| TI TMS320DM365 ZCE IBIS MODEL
[IBIS Ver]   4.0
[File Name]   sprm354.ibs
[File Rev]   1.02
[Date]   August 12, 2010
[Source]   From silicon level SPICE model at Texas Instruments Inc.,
[Notes]   -RevA   Added DDR IBIS info.
		-RevB 	Updated/fixed DDR IBIS info.
   -RevC   Remove a unnecessary note.
[Disclaimer] Please be aware that in the absence of a written agreement,
   Texas Instruments (TI) assumes no liability for: 1) the
   accuracy of the IBIS models provided to your company, 2) the
   proper functioning of these IBIS models in your design or for
   any resulting applications, or; 3) infringement of patents,
   copyrights, or intellectual property rights resulting from
   your use of these IBIS models. TI provides IBIS models as a
   service to our customers and therefore reserves the right to
   limit distribution of the IBIS models.
[Copyright]   Property of Texas Instruments Incorporated. Unauthorized
   reproduction and/or distribution is strictly prohibited. This
   product is protected under copyright law and trade secret law
   as an unpublished work. Copyright (C) 2008, Texas Instruments
   Incorporated, all rights reserved. These commodities are under
   the U.S. Government distribution license control. As such,
   they are not to be re-exported without the prior approval of
   the U.S. Department of Commerce.
| Component   DM365
[Component]   DM365
[Manufacturer]   Texas Instruments
[Package]
| variable   typ   min   max
R_pkg   2.50E-01   2.85E-03   3.42E-01
L_pkg   3.37E-09   8.62E-11   5.01E-09
C_pkg   9.39E-13   4.32E-13   3.43E-11
[Pin] signal_name   model_name   R_pin   L_pin   C_pin
W19   VSS   GND   2.85E-03   8.62E-11   3.43E-11
A1   RSV0   NC   2.88E-01   4.46E-09   4.90E-13
E5   VDD18_SLD0   POWER   5.60E-02   1.13E-09   7.80E-13
D4   VDDRAM   NC   2.37E-01   3.20E-09   7.66E-13
B3   GIO6   BC1833DV65ATHYPBFZP   2.43E-01   3.73E-09   7.84E-13
H6   VDDS33   POWER   8.08E-03   1.69E-10   1.01E-11
A3   GIO7   BC1833DV65ATHYPBFZP   3.13E-01   4.61E-09   8.76E-13
A2   GIO8   BC1833DV65ATHYPBFZP   3.06E-01   4.77E-09   6.55E-13
C2   GIO9   BC1833DV65ATHYPBFZP   2.29E-01   3.51E-09   8.41E-13
B2   GIO10   BC1833DV65ATHYPBFZP   3.19E-01   4.70E-09   7.26E-13
G6   CVDD   POWER   5.00E-03   1.20E-10   2.07E-11
B1   GIO11   BC1833DV65ATHYPBFZP   3.18E-01   4.90E-09   5.92E-13
C1   GIO12   BC1833DV65ATHYPBFZP   2.88E-01   4.22E-09   5.60E-13
D3   GIO13   BC1833DV65ATHYPBFZP   2.21E-01   3.18E-09   7.81E-13
D1   GIO14   BC1833DV65ATHYPBFZP   2.85E-01   4.00E-09   4.66E-13
D2   GIO15   BC1833DV65ATHYPBFZP   2.85E-01   3.85E-09   5.44E-13
E1   GIO16   BC1833DV65ATHYPBFZP   2.36E-01   3.69E-09   5.56E-13
E4   GIO17   BC1833DV65ATHYPBFZP   2.26E-01   3.16E-09   6.86E-13
E2   GIO18   BC1833DV65ATHYPBFZP   2.99E-01   3.96E-09   6.09E-13
E3   GIO19   BC1833DV65ATHYPBFZP   2.97E-01   3.86E-09   6.67E-13
F1   GIO20   BC1833DV65ATHYPBFZP   2.76E-01   4.04E-09   6.21E-13
F3   GIO21   BC1833DV65ATHYPBFZP   2.19E-01   2.93E-09   6.69E-13
F2   RTCK   BC1833DV65ATHYPBFZP   2.63E-01   3.42E-09   5.45E-13
F4   TCK   BC1833DV65ATHYPBFZP   2.31E-01   3.14E-09   7.64E-13
F5   TDI   BC1833DV65ATHYPBFZP   2.42E-01   3.30E-09   9.98E-13
G4   TDO   BC1833DV65ATHYPBFZP   2.22E-01   2.99E-09   7.49E-13
G2   TMS   BC1833DV65ATHYPBFZP   2.81E-01   3.79E-09   6.26E-13
G5   EMU0   BC1833DV65ATHYPBFZP   2.35E-01   3.19E-09   8.20E-13
H4   EMU1   BC1833DV65ATHYPBFZP   2.92E-01   3.68E-09   7.83E-13
H5   TRSTN   BC1833DV65ATHYPBFZP   3.18E-01   3.89E-09   8.80E-13
H3   RESETN   NC   2.10E-01   2.68E-09   6.04E-13
G1   RTCXI   NC   2.23E-01   3.66E-09   6.19E-13
H2   VSS_32K   GND   1.99E-01   2.72E-09   9.76E-13
H1   RTCXO   NC   2.11E-01   3.30E-09   5.11E-13
J6   VDD12_PRTCSS   POWER   3.50E-02   7.90E-10   2.34E-12
J3   PWCTRIO0   BQ1865ACTHYPOFFFBPB   2.79E-01   3.43E-09   6.80E-13
J2   PWCTRIO1   BQ1865ACTHYPOFFFBPB   2.53E-01   3.27E-09   5.62E-13
K6   VDD18_PRTCSS   POWER   6.00E-02   1.04E-09   1.13E-12
J1   PWCTRIO2   BQ1865ACTHYPOFFFBPB   2.57E-01   3.58E-09   5.01E-13
J5   PWCTRIO3   BQ1865ACTHYPOFFFBPB   2.54E-01   3.40E-09   8.60E-13
J4   PWCTRIO4   BQ1865ACTHYPOFFFBPB   1.06E-01   1.76E-09   6.11E-13
K5   PWCTRIO5   BQ1865ACTHYPOFFFBPB   2.54E-01   3.22E-09   7.91E-13
K4   PWCTRIO6   BQ1865ACTHYPOFFFBPB   2.08E-01   2.63E-09   7.15E-13
K2   PWCTRO0   BQ1865ACTHYPOFFFBPB   2.51E-01   3.27E-09   5.84E-13
L5   PWCTRO1   BQ1865ACTHYPOFFFBPB   2.42E-01   3.14E-09   8.14E-13
L4   PWCTRO2   BQ1865ACTHYPOFFFBPB   2.22E-01   2.87E-09   7.19E-13
L3   PWCTRO3   BQ1865ACTHYPOFFFBPB   2.12E-01   2.73E-09   5.88E-13
M3   PWRST   BQ1865ACTHYPOFFFBPB   1.25E-01   2.36E-09   6.13E-13
M2   PWRCNTON   BQ1865ACTHYPOFFFBPB   2.12E-01   2.89E-09   6.38E-13
K1   MXO1   NC   2.25E-01   3.75E-09   6.17E-13
L2   VSS_27M   GND   2.33E-01   4.03E-09   8.90E-13
L1   MXI1   NC   2.23E-01   3.57E-09   5.75E-13
L6   VDDMXI   POWER   1.22E-01   1.99E-09   8.19E-13
N4   VDDA18_PLL   POWER   1.31E-01   2.34E-09   7.26E-13
M4   VSSA   GND   1.15E-01   1.72E-09   6.70E-13
M1   USB_ID   NC   2.63E-01   3.87E-09   5.58E-13
N2   USB_VBUS   NC   2.57E-01   3.25E-09   5.62E-13
M5   VDDA12LDO_USB  POWER   1.17E-01   1.57E-09   7.09E-13
N5   VDDA18_USB   POWER   1.11E-01   1.56E-09   7.34E-13
P2   VSSAUSB_USB   GND   1.27E-01   2.49E-09   5.78E-13
N1   USB_DP   USB_DATA_DP   2.15E-01   3.53E-09   5.99E-13
P1   USB_DM   USB_DATA_DM   2.16E-01   3.52E-09   5.17E-13
P3   VSSA33_USB   GND   1.13E-01   2.14E-09   6.26E-13
P4   VDDA33_USB   GND   1.08E-01   1.81E-09   7.69E-13
R4   RSV2   NC   2.90E-01   3.72E-09   7.56E-13
R3   VPP   POWER   1.19E-01   2.41E-09   8.21E-13
R1   RSV1   NC   2.58E-01   3.80E-09   4.76E-13
R2   GIO22   BC1833DV65ATHYPBFZP   2.58E-01   3.32E-09   5.57E-13
V2   GIO23   BC1833DV65ATHYPBFZP   3.04E-01   4.25E-09   7.73E-13
T3   GIO24   BC1833DV65ATHYPBFZP   2.05E-01   3.12E-09   5.75E-13
T1   GIO25   BC1833DV65ATHYPBFZP   2.68E-01   3.80E-09   4.77E-13
U1   GIO26   BC1833DV65ATHYPBFZP   2.76E-01   4.23E-09   5.58E-13
T2   GIO27   BC1833DV65ATHYPBFZP   2.64E-01   3.41E-09   5.21E-13
V1   GIO28   BC1833DV65ATHYPBFZP   2.83E-01   4.30E-09   5.37E-13
U2   GIO29   BC1833DV65ATHYPBFZP   2.69E-01   3.62E-09   5.05E-13
T4   GIO30   BC1833DV65ATHYPBFZP   1.02E-01   1.93E-09   7.40E-13
U4   GIO31   BC1833DV65ATHYPBFZP   1.37E-01   2.47E-09   8.39E-13
W2   GIO32   BC1833DV65ATHYPBFZP   2.98E-01   4.29E-09   4.90E-13
V3   GIO33   BC1833DV65ATHYPBFZP   2.09E-01   3.06E-09   7.00E-13
V4   GIO34   BC1833DV65ATHYPBFZP   2.95E-01   3.73E-09   6.31E-13
W3   GIO35   BC1833DV65ATHYPBFZP   2.91E-01   4.06E-09   4.69E-13
W4   GIO36   BC1833DV65ATHYPBFZP   2.55E-01   3.95E-09   5.93E-13
T5   GIO37   BC1833DV65ATHYPBFZP   2.76E-01   3.86E-09   9.59E-13
V5   GIO38   BC1833DV65ATHYPBFZP   3.11E-01   4.41E-09   6.63E-13
R5   GIO39   BC1833DV65ATHYPBFZP   2.55E-01   3.75E-09   7.73E-13
U5   GIO40   BC1833DV65ATHYPBFZP   2.96E-01   3.70E-09   6.51E-13
W5   GIO41   BC1833DV65ATHYPBFZP   2.84E-01   4.01E-09   5.64E-13
R6   GIO42   BC1833DV65ATHYPBFZP   2.78E-01   4.08E-09   8.81E-13
T6   GIO43   BC1833DV65ATHYPBFZP   2.34E-01   3.14E-09   6.91E-13
W6   DDR_DQM1   BSSTL18TCSCGPBFZ   2.43E-01   3.86E-09   5.87E-13
V6   DDR_DQ15   BSSTL18TCSCGPBFZ   2.17E-01   3.02E-09   5.03E-13
N9   VDD18_DDR   POWER   1.01E-02   2.26E-10   4.96E-12
V7   DDR_DQ14   BSSTL18TCSCGPBFZ   2.79E-01   3.56E-09   6.03E-13
R7   DDR_DQ13   BSSTL18TCSCGPBFZ   2.64E-01   3.80E-09   9.68E-13
W7   DDR_DQ12   BSSTL18TCSCGPBFZ   2.75E-01   3.97E-09   5.44E-13
U6   DDR_DQSN1   BSSTL18TCSCGPBFZ   2.30E-01   3.20E-09   6.51E-13
T7   DDR_DQS1   BSSTL18TCSCGPBFZ   2.29E-01   3.15E-09   7.15E-13
V8   DDR_DQ11   BSSTL18TCSCGPBFZ   2.76E-01   3.51E-09   6.02E-13
R8   DDR_DQ10   BSSTL18TCSCGPBFZ   2.41E-01   3.25E-09   9.30E-13
U8   DDR_DQ9   BSSTL18TCSCGPBFZ   2.90E-01   3.61E-09   6.56E-13
W8   DDR_DQ8   BSSTL18TCSCGPBFZ   2.66E-01   3.74E-09   4.78E-13
T9   DDR_DQGATE1   BSSTL18TCSCGPBFZ   2.11E-01   2.63E-09   6.77E-13
T8   DDR_DQGATE0   BSSTL18TCSCGPBFZ   3.00E-01   4.03E-09   8.02E-13
R9   DDR_DQ7   BSSTL18TCSCGPBFZ   2.43E-01   3.56E-09   8.33E-13
W9   DDR_DQ6   BSSTL18TCSCGPBFZ   2.51E-01   3.45E-09   4.75E-13
V9   DDR_DQ5   BSSTL18TCSCGPBFZ   2.65E-01   3.42E-09   6.43E-13
W10   DDR_DQ4   BSSTL18TCSCGPBFZ   2.07E-01   3.27E-09   5.20E-13
U9   DDR_DQSN0   BSSTL18TCSCGPBFZ   2.23E-01   2.89E-09   6.29E-13
T10   DDR_DQS0   BSSTL18TCSCGPBFZ   2.21E-01   2.89E-09   7.26E-13
V10   DDR_DQ3   BSSTL18TCSCGPBFZ   2.56E-01   3.21E-09   6.03E-13
R11   DDR_PADREFP   NC   1.54E-01   2.70E-09   8.40E-13
R10   DDR_DQ2   BSSTL18TCSCGPBFZ   2.43E-01   3.20E-09   7.81E-13
V11   DDR_DQ1   BSSTL18TCSCGPBFZ   2.70E-01   3.61E-09   5.89E-13
U11   DDR_DQ0   BSSTL18TCSCGPBFZ   2.78E-01   3.40E-09   6.81E-13
T11   DDR_DQM0   BSSTL18TCSCGPBFZ   2.98E-01   3.71E-09   8.31E-13
P11   DDR_VREF   NC   1.66E-01   2.83E-09   1.06E-12
W11   DDR_CLK   BSSTL18TCSCGPBFZ   2.08E-01   3.23E-09   5.21E-13
W12   DDR_CLKN   BSSTL18TCSCGPBFZ   2.04E-01   3.11E-09   5.33E-13
T12   DDR_CSN   BSSTL18TCSCGPBFZ   2.17E-01   2.86E-09   7.02E-13
V12   DDR_CASN   BSSTL18TCSCGPBFZ   2.42E-01   3.47E-09   6.40E-13
R13   DDR_CKE   BSSTL18TCSCGPBFZ   2.45E-01   3.52E-09   8.95E-13
U12   DDR_RASN   BSSTL18TCSCGPBFZ   2.02E-01   2.64E-09   6.24E-13
W13   DDR_WEN   BSSTL18TCSCGPBFZ   2.22E-01   3.53E-09   5.83E-13
V13   DDR_BA2   BSSTL18TCSCGPBFZ   2.93E-01   3.67E-09   7.31E-13
T13   DDR_BA1   BSSTL18TCSCGPBFZ   2.08E-01   2.82E-09   7.62E-13
W14   DDR_BA0   BSSTL18TCSCGPBFZ   2.58E-01   3.73E-09   5.69E-13
U14   DDR_A0   BSSTL18TCSCGPBFZ   2.81E-01   3.68E-09   6.60E-13
V14   DDR_A1   BSSTL18TCSCGPBFZ   2.57E-01   3.32E-09   5.93E-13
W15   DDR_A2   BSSTL18TCSCGPBFZ   2.60E-01   3.98E-09   5.89E-13
T14   DDR_A3   BSSTL18TCSCGPBFZ   2.10E-01   2.92E-09   6.92E-13
U15   DDR_A4   BSSTL18TCSCGPBFZ   2.80E-01   3.77E-09   6.17E-13
V15   DDR_A5   BSSTL18TCSCGPBFZ   2.61E-01   3.50E-09   5.56E-13
W16   DDR_A6   BSSTL18TCSCGPBFZ   2.72E-01   4.15E-09   5.80E-13
T15   DDR_A7   BSSTL18TCSCGPBFZ   2.04E-01   2.84E-09   6.44E-13
W17   DDR_A8   BSSTL18TCSCGPBFZ   2.84E-01   4.59E-09   6.29E-13
U16   DDR_A9   BSSTL18TCSCGPBFZ   2.95E-01   3.98E-09   7.35E-13
V16   DDR_A10   BSSTL18TCSCGPBFZ   2.67E-01   3.60E-09   6.04E-13
W18   DDR_A11   BSSTL18TCSCGPBFZ   2.95E-01   4.75E-09   6.09E-13
V17   DDR_A12   BSSTL18TCSCGPBFZ   2.20E-01   3.60E-09   6.91E-13
T16   DDR_A13   BSSTL18TCSCGPBFZ   2.41E-01   3.43E-09   8.11E-13
P14   VDD_AEMIF1_18_33  POWER   2.34E-02   4.32E-10   2.51E-12
V18   EM_A13   BC1833DV50BTHYPBFZP   2.57E-01   4.37E-09   6.53E-13
U18   EM_A12   BC1833DV50BTHYPBFZP   2.84E-01   3.69E-09   6.05E-13
V19   EM_A11   BC1833DV50BTHYPBFZP   2.63E-01   3.81E-09   5.49E-13
U19   EM_A10   BC1833DV50BTHYPBFZP   3.14E-01   4.74E-09   6.55E-13
T18   EM_A9   BC1833DV50BTHYPBFZP   2.94E-01   3.89E-09   7.31E-13
T19   EM_A8   BC1833DV50BTHYPBFZP   3.20E-01   4.78E-09   6.82E-13
T17   EM_A7   BC1833DV50BTHYPBFZP   2.94E-01   3.81E-09   6.87E-13
R18   EM_A6   BC1833DV50BTHYPBFZP   2.89E-01   3.70E-09   6.69E-13
R16   EM_A5   BC1833DV50BTHYPBFZP   1.80E-01   3.37E-09   8.13E-13
R19   EM_A4   BC1833DV50BTHYPBFZP   3.03E-01   4.53E-09   6.45E-13
R15   EM_A3   BC1833DV50BTHYPBFZP   3.27E-01   4.36E-09   8.36E-13
R17   EM_BA1   BC1833DV50BTHYPBFZP   2.97E-01   4.20E-09   7.34E-13
P17   EM_BA0   BC1833DV50BTHYPBFZP   3.01E-01   3.95E-09   7.23E-13
P18   EM_D15   BC1833DV50BTHYPBFZP   2.96E-01   4.04E-09   6.61E-13
P16   EM_D14   BC1833DV50BTHYPBFZP   2.28E-01   3.02E-09   6.96E-13
P19   EM_D13   BC1833DV50BTHYPBFZP   2.72E-01   3.86E-09   5.76E-13
P15   EM_D12   BC1833DV50BTHYPBFZP   3.14E-01   4.26E-09   8.08E-13
N16   EM_D11   BC1833DV50BTHYPBFZP   2.46E-01   3.17E-09   7.42E-13
N18   EM_D10   BC1833DV50BTHYPBFZP   2.26E-01   3.06E-09   6.33E-13
N19   EM_D9   BC1833DV50BTHYPBFZP   2.67E-01   3.84E-09   5.65E-13
N15   EM_D8   BC1833DV50BTHYPBFZP   2.49E-01   3.50E-09   8.22E-13
M17   EM_CE0   BC1833DV50BTHYPBFZP   2.82E-01   3.66E-09   7.06E-13
M16   EM_ADV   BC1833DV50BTHYPBFZP   2.45E-01   3.15E-09   7.36E-13
M15   EM_CLK   BC1833DV40CTHYPBFZP   2.59E-01   3.41E-09   7.66E-13
M18   EM_A2   BC1833DV50BTHYPBFZP   2.18E-01   2.92E-09   5.52E-13
K14   VDD_AEMIF2_18_33 POWER   3.81E-02   5.98E-10   1.66E-12
M19   EM_A1   BC1833DV50BTHYPBFZP   2.42E-01   3.69E-09   5.48E-13
L17   EM_A0   BC1833DV50BTHYPBFZP   2.72E-01   3.41E-09   6.46E-13
L16   EM_D7   BC1833DV50BTHYPBFZP   2.89E-01   4.53E-09   7.99E-13
L18   EM_D6   BC1833DV50BTHYPBFZP   2.82E-01   3.74E-09   5.84E-13
L19   EM_D5   BC1833DV50BTHYPBFZP   2.57E-01   3.63E-09   5.10E-13
L15   EM_D4   BC1833DV50BTHYPBFZP   2.59E-01   3.48E-09   7.99E-13
K15   EM_D3   BC1833DV50BTHYPBFZP   2.58E-01   3.32E-09   8.09E-13
K19   EM_D2   BC1833DV50BTHYPBFZP   2.32E-01   3.54E-09   5.46E-13
K16   EM_D1   BC1833DV50BTHYPBFZP   2.29E-01   2.93E-09   7.80E-13
K18   EM_D0   BC1833DV50BTHYPBFZP   2.71E-01   3.36E-09   6.88E-13
J17   EM_CE1   BC1833DV50BTHYPBFZP   2.71E-01   3.39E-09   7.15E-13
J15   EM_WE   BC1833DV50BTHYPBFZP   2.59E-01   3.41E-09   8.14E-13
J19   EM_OE   BC1833DV50BTHYPBFZP   2.14E-01   3.26E-09   5.61E-13
J18   EM_WAIT   BC1833DV50BTHYPBFZP   2.15E-01   2.89E-09   5.81E-13
J16   MMCSD0_CLK   BC1833DV65ATHYPBFZP   2.37E-01   3.07E-09   7.18E-13
H15   MMCSD0_CMD   BC1833DV65ATHYPBFZP   3.43E-01   4.63E-09   8.58E-13
H16   MMCSD0_DATA3   BC1833DV65ATHYPBFZP   2.36E-01   3.31E-09   7.67E-13
H17   MMCSD0_DATA2   BC1833DV65ATHYPBFZP   2.88E-01   3.69E-09   6.84E-13
H19   MMCSD0_DATA1   BC1833DV65ATHYPBFZP   2.36E-01   3.61E-09   5.20E-13
H18   MMCSD0_DATA0   BC1833DV65ATHYPBFZP   2.79E-01   3.88E-09   5.96E-13
G15   HSYNC   BC1833DV50BTHYPBFZP   3.09E-01   3.99E-09   7.84E-13
G18   VSYNC   BC1833DV50BTHYPBFZP   2.61E-01   3.38E-09   5.49E-13
G16   YOUT7   BC1833DV50BTHYPBFZP   2.25E-01   3.04E-09   6.96E-13
G19   YOUT6   BC1833DV50BTHYPBFZP   2.59E-01   3.65E-09   4.77E-13
F15   YOUT5   BC1833DV50BTHYPBFZP   3.13E-01   4.24E-09   8.12E-13
F18   YOUT4   BC1833DV50BTHYPBFZP   2.78E-01   3.92E-09   5.75E-13
F16   YOUT3   BC1833DV50BTHYPBFZP   2.41E-01   3.17E-09   7.30E-13
F19   YOUT2   BC1833DV50BTHYPBFZP   2.65E-01   3.75E-09   4.82E-13
F17   YOUT1   BC1833DV50BTHYPBFZP   2.35E-01   3.13E-09   6.50E-13
E16   YOUT0   BC1833DV50BTHYPBFZP   2.67E-01   3.71E-09   7.82E-13
E18   COUT7   BC1833DV50BTHYPBFZP   2.24E-01   3.24E-09   5.49E-13
E19   COUT6   BC1833DV50BTHYPBFZP   2.76E-01   3.94E-09   4.87E-13
E15   COUT5   BC1833DV50BTHYPBFZP   2.56E-01   3.62E-09   7.50E-13
E17   COUT4   BC1833DV50BTHYPBFZP   2.89E-01   3.88E-09   6.41E-13
D16   COUT3   BC1833DV50BTHYPBFZP   2.44E-01   3.37E-09   6.09E-13
D19   COUT2   BC1833DV50BTHYPBFZP   2.53E-01   3.90E-09   5.07E-13
D18   COUT1   BC1833DV50BTHYPBFZP   2.38E-01   3.48E-09   5.04E-13
D17   COUT0   BC1833DV50BTHYPBFZP   2.86E-01   3.61E-09   5.76E-13
C19   LCD_OE   BC1833DV50BTHYPBFZP   2.94E-01   4.21E-09   5.20E-13
C18   FIELD   BC1833DV50BTHYPBFZP   2.87E-01   3.64E-09   5.75E-13
B19   EXTCLK   BC1833DV50BTHYPBFZP   3.06E-01   4.38E-09   4.59E-13
B18   VCLK   BC1833DV50BTHYPBFZP   3.03E-01   3.85E-09   6.48E-13
F12   VDD_ISIF18_33  POWER   3.12E-02   5.85E-10   2.92E-12
B17   CIN0   BC1833DV50BTHYPBFZP   2.78E-01   3.58E-09   5.46E-13
A18   CIN1   BC1833DV50BTHYPBFZP   2.76E-01   4.05E-09   5.04E-13
C16   CIN2   BC1833DV50BTHYPBFZP   2.03E-01   2.69E-09   6.55E-13
A17   CIN3   BC1833DV50BTHYPBFZP   2.69E-01   3.82E-09   4.32E-13
A16   CIN4   BC1833DV50BTHYPBFZP   2.74E-01   3.83E-09   5.12E-13
B16   CIN5   BC1833DV50BTHYPBFZP   2.80E-01   3.63E-09   5.82E-13
C15   CIN6   BC1833DV50BTHYPBFZP   2.94E-01   3.77E-09   6.83E-13
A15   CIN7   BC1833DV50BTHYPBFZP   2.58E-01   3.60E-09   5.00E-13
D15   YIN0   BC1833DV50BTHYPBFZP   2.28E-01   3.46E-09   7.43E-13
D14   YIN1   BC1833DV50BTHYPBFZP   2.92E-01   3.71E-09   7.38E-13
B15   YIN2   BC1833DV50BTHYPBFZP   2.99E-01   3.97E-09   7.27E-13
A14   YIN3   BC1833DV50BTHYPBFZP   2.49E-01   3.40E-09   4.96E-13
C14   HD   BC1833DV50BTHYPBFZP   2.82E-01   3.65E-09   6.61E-13
B14   VD   BC1833DV50BTHYPBFZP   2.58E-01   3.38E-09   5.53E-13
E13   C_WE_FIELD   BC1833DV50BTHYPBFZP   2.32E-01   3.03E-09   7.62E-13
D13   PCLK   BC1833DV50BTHYPBFZP   2.97E-01   3.89E-09   7.64E-13
D12   YIN4   BC1833DV50BTHYPBFZP   2.93E-01   3.61E-09   7.35E-13
B13   YIN5   BC1833DV50BTHYPBFZP   2.60E-01   3.27E-09   5.38E-13
A13   YIN6   BC1833DV50BTHYPBFZP   2.51E-01   3.30E-09   5.10E-13
C12   YIN7   BC1833DV50BTHYPBFZP   2.71E-01   3.41E-09   6.51E-13
E12   VDDA12_DAC   POWER   1.15E-01   1.58E-09   7.96E-13
F11   VSSA12_DAC   GND   1.29E-01   2.21E-09   9.42E-13
B12   COMPY   NC   2.58E-01   3.19E-09   6.11E-13
D10   VDDA18_DAC   POWER   4.10E-02   9.40E-10   1.06E-12
A12   COMPPB   NC   2.44E-01   3.14E-09   5.45E-13
E11   VSSA18_DAC   GND   4.10E-02   6.90E-10   1.24E-12
C11   COMPPR   NC   2.67E-01   3.28E-09   6.79E-13
A11   IREF   NC   2.39E-01   3.26E-09   4.50E-13
D11   VREF   NC   2.68E-01   3.77E-09   7.24E-13
B11   IDACOUT   NC   2.61E-01   3.30E-09   5.66E-13
B10   VFB   NC   2.51E-01   3.10E-09   5.56E-13
A10   TVOUT   NC   2.40E-01   3.30E-09   5.09E-13
E10   VDDA33_VC   POWER   6.60E-02   1.29E-09   8.61E-13
A9   SPN   NC   1.95E-01   2.89E-09   5.09E-13
B9   SPP   NC   1.97E-01   2.68E-09   5.10E-13
D9   VSSA33_VC   GND   5.60E-02   1.19E-09   7.06E-13
C9   LINEO   NC   2.73E-01   3.39E-09   6.60E-13
E9   VDDA18_VC   POWER   1.19E-01   1.86E-09   7.77E-13
A8   VCOM   NC   2.38E-01   3.27E-09   5.09E-13
F9   VSSA18_VC   GND   1.30E-01   2.33E-09   9.57E-13
C8   MICIN   NC   2.65E-01   3.26E-09   6.49E-13
B8   MICIP   NC   2.61E-01   3.26E-09   6.21E-13
E8   ADC_CH0   NC   1.27E-01   2.07E-09   8.94E-13
B7   ADC_CH1   NC   2.71E-01   3.38E-09   6.28E-13
G9   VDDA18V_ADC   POWER   8.20E-02   2.30E-09   1.32E-12
A7   ADC_CH2   NC   2.51E-01   3.49E-09   5.11E-13
F8   VSSAV_ADC   GND   6.40E-02   1.33E-09   1.28E-12
D7   ADC_CH4   NC   2.91E-01   3.66E-09   9.51E-13
D8   ADC_CH3   NC   2.06E-01   2.68E-09   7.22E-13
A6   ADC_CH5   NC   2.51E-01   3.47E-09   4.89E-13
E7   GIO44   BC1833DV65ATHYPBFZP   3.22E-01   4.22E-09   8.45E-13
B6   GIO45   BC1833DV65ATHYPBFZP   2.83E-01   3.98E-09   6.26E-13
C6   GIO47   BC1833DV65ATHYPBFZP   2.95E-01   3.69E-09   7.19E-13
E6   GIO46   BC1833DV65ATHYPBFZP   2.37E-01   3.07E-09   7.92E-13
A5   GIO48   BC1833DV65ATHYPBFZP   2.68E-01   3.88E-09   5.90E-13
B5   GIO0   BC1833DV65ATHYPBFZP   2.73E-01   3.44E-09   5.81E-13
D5   GIO49   BC1833DV65ATHYPBFZP   2.16E-01   2.91E-09   6.72E-13
D6   GIO1   BC1833DV65ATHYPBFZP   3.42E-01   4.49E-09   9.38E-13
C5   GIO3   BC1833DV65ATHYPBFZP   2.49E-01   3.34E-09   7.21E-13
C4   GIO2   BC1833DV65ATHYPBFZP   2.01E-01   2.67E-09   6.01E-13
A4   GIO4   BC1833DV65ATHYPBFZP   3.08E-01   4.59E-09   6.56E-13
B4   GIO5   BC1833DV65ATHYPBFZP   3.36E-01   5.09E-09   7.27E-13|
[Diff Pin] inv_pin vdiff tdelay_typ tdelay_min tdelay_max
N1   P1   0   1nS   NA   NA
T7   U6   0   0   NA   NA
T10   U9   0   0   NA   NA
W11   W12   0   0   NA   NA
[Model Selector] BC1833DV40CTHYPBFZP
BC40C_PI_1P8  Cell operated at 1.8(nom)
|BC1833DV40CTHYPBFZP_PI_1P8; BUFFER IN NORMAL MODE WITH PULLUP AND
|PULLDOWN OFF
BC40C_PI_3P3  Cell operated at 3.3(nom)
|BC1833DV40CTHYPBFZP_PI_3P3; BUFFER IN NORMAL MODE WITH PULLUP AND
|PULLDOWN OFF [Model Selector] BC3350BSHYPUFZP18
[Model Selector] BC1833DV50BTHYPBFZP
BC50B_!PI_LOW_1P8  Cell operated at 1.8(nom)
|BC1833DV50BTHYPBFZP_!PI_LOW_1P8; BUFFER WITH WEAK_PULLDOWN_ON NOMI
|NAL CURRENT OF 100UA WHEN PAD=VDDS
BC50B_!PI_HIGH_1P8  Cell operated at 1.8(nom)
|BC1833DV50BTHYPBFZP_!PI_HIGH_1P8; BUFFER WITH WEAK_PULLUP_ON NOMIN
|AL CURRENT OF 100UA WHEN PAD=0
BC50B_PI_1P8  Cell operated at 1.8(nom)
|BC1833DV50BTHYPBFZP_PI_1P8; BUFFER IN NORMAL MODE WITH PULLUP AND
|PULLDOWN OFF
BC50B_!PI_LOW_3P3  Cell operated at 3.3(nom)
|BC1833DV50BTHYPBFZP_!PI_LOW_3P3; BUFFER WITH WEAK_PULLDOWN_ON NOMI
|NAL CURRENT OF 100UA WHEN PAD=VDDS
BC50B_!PI_HIGH_3P3  Cell operated at 3.3(nom)
|BC1833DV50BTHYPBFZP_!PI_HIGH_3P3; BUFFER WITH WEAK_PULLUP_ON NOMIN
|AL CURRENT OF 100UA WHEN PAD=0
BC50B_PI_3P3  Cell operated at 3.3(nom)
|BC1833DV50BTHYPBFZP_PI_3P3; BUFFER IN NORMAL MODE WITH PULLUP AND
|PULLDOWN OFF
[Model Selector] BC1833DV65ATHYPBFZP
BC65A_!PI_LOW_3P3  Cell operated at 3.3(nom)
|BC1833DV65ATHYPBFZP_!PI_LOW_3P3; BUFFER WITH WEAK_PULLDOWN_ON NOMI
|NAL CURRENT OF 100UA WHEN PAD=VDDS
BC65A_!PI_HIGH_3P3  Cell operated at 3.3(nom)
|BC1833DV65ATHYPBFZP_!PI_HIGH_3P3; BUFFER WITH WEAK_PULLUP_ON NOMIN
|AL CURRENT OF 100UA WHEN PAD=0
BC65A_PI_3P3  Cell operated at 3.3(nom)
|BC1833DV65ATHYPBFZP_PI_3P3; BUFFER IN NORMAL MODE WITH PULLUP AND
|PULLDOWN OFF
[Model Selector] BQ1865ACTHYPOFFFBPB
HYPOFFFBPB_PD_PU_1P8  Cell operated at 1.8(nom)
|BQ1865ACTHYPOFFFBPB_PD_PU_1P8BUFFER IN NORMAL MODE WITH PULLUP/PULLDOWN OF
|F
YPOFFFBPB_PD_PU_1P12  Cell operated at 1.12(nom)
|BQ1865ACTHYPOFFFBPB_PD_PU_1P12; BUFFER IN NORMAL MODE WITH PULLUP/PULLDOWN
| OFF
[Model Selector] USB_DATA_DP
hs_dp   usb dp for high speed mode
fs_dp   usb dp for full speed mode
[Model Selector] USB_DATA_DM
hs_dm   usb dm for high speed mode
fs_dm   usb dm for full speed mode
[Model Selector] BSSTL18TCSCGPBFZ
|CELL OPERATING AT TWO VOLTAGES.1.5V/1.8V-DUAL SUPPLY
|SR0 IS SLEW RATE CONTROL BIT WHICH DECIDES THE MODE OF OPERATION
|T0 AND T1 ARE TERMINATION BITS WHICH CAUSE NO,HALF,FULL TERMINATION
|NO TERMINATION WHEN T0=0 WHEN T1=0
|HALF TERMINATION WHEN T0=1 WHEN T1=0
|FULL TERMINATION WHEN T0=0 WHEN T1=1
|SSTL RECIEVER MODE WHEN CMOSEN = 0
|LVCMOS RECIEVER MODE WHEN CMOSEN = 1
HALF_TERM_SSTL_1P8  Cell operated at 1.8(nom)
|HALF_TERM_SSTL_1P8
|BUFFER OPERATING UNDER HALF TERMINATION MODE AND SSTL RECIVER MODE WITH
| 1.8V SUPPLY WITH +/-10% VARIATION
HALF_TERM_LVCMOS_1P8  Cell operated at 1.8(nom)
|HALF_TERM_LVCMOS_1P8
|BUFFER OPERATING UNDER HALF TERMINATION MODE AND LVCMOS RECIVER MODE WITH
| 1.8V SUPPLY WITH +/-10% VARIATION
NOSR0_NOTERM_1P8  Cell operated at 1.8(nom)
|NOSR0_NOTERM_1P8
|BUFFER OPERATING AT FAST MODE WITH 1.8V SUPPLY WITH +/-10% VARIATION
SR0_NOTERM_1P8  Cell operated at 1.8(nom)
|SR0_NOTERM_1P8
|BUFFER OPERATING AT SLOW MODE WITH 1.8V SUPPLY WITH +/-10% VARIATION
FULL_TERM_SSTL_1P8  Cell operated at 1.8(nom)
|FULL_TERM_SSTL_1P8
|BUFFER OPERATING UNDER FULL TERMINATION MODE AND SSTL RECIVER MODE WITH
| 1.8V SUPPLY WITH +/-10% VARIATION
NO_TERM_LVCMOS_1P8  Cell operated at 1.8(nom)
|NO_TERM_LVCMOS_1P8
|BUFFER OPERATING UNDER NO TERMINATION MODE AND LVCMOS RECIVER MODE WITH
| 1.8V SUPPLY WITH +/-10% VARIATION
FULL_TERM_LVCMOS_1P8  Cell operated at 1.8(nom)
|FULL_TERM_LVCMOS_1P8
|BUFFER OPERATING UNDER FULL TERMINATION MODE AND LVCMOS RECIVER MODE WITH
| 1.8V SUPPLY WITH +/-10% VARIATION
NO_TERM_SSTL_1P8  Cell operated at 1.8(nom)
|NO_TERM_SSTL_1P8
|BUFFER OPERATING UNDER NO TERMINATION MODE AND SSTL RECIVER MODE WITH
| 1.8V SUPPLY WITH +/-10% VARIATION
HALF_TERM_SSTL_1P5  Cell operated at 1.5(nom)
|HALF_TERM_SSTL_1P5
|BUFFER OPERATING UNDER HALF TERMINATION MODE AND SSTL RECIVER MODE WITH
| 1.5V SUPPLY WITH +/-10% VARIATION
NOSR0_NOTERM_1P5  Cell operated at 1.5(nom)
|NOSR0_NOTERM_1P5
|BUFFER OPERATING AT FAST MODE WITH 1.5V SUPPLY WITH +/-10% VARIATION
SR0_NOTERM_1P5  Cell operated at 1.5(nom)
|SR0_NOTERM_1P5
|BUFFER OPERATING AT SLOW MODE WITH 1.5V SUPPLY WITH +/-10% VARIATION
FULL_TERM_SSTL_1P5  Cell operated at 1.5(nom)
|FULL_TERM_SSTL_1P5
|BUFFER OPERATING UNDER FULL TERMINATION MODE AND SSTL RECIVER MODE WITH
| 1.5V SUPPLY WITH +/-10% VARIATION
NO_TERM_SSTL_1P5  Cell operated at 1.5(nom)
|NO_TERM_SSTL_1P5
|BUFFER OPERATING UNDER NO TERMINATION MODE AND SSTL RECIVER MODE WITH
| 1.5V SUPPLY WITH +/-10% VARIATION
LF_TERM_SSTL_0.1_1P8  Cell operated at 1.8(nom)
|HALF_TERM_SSTL_0.1_1P8
|BUFFER OPERATING UNDER HALF TERMINATION MODE AND SSTL RECIVER MODE WITH
| 1.8V SUPPLY WITH +/-0.1V VARIATION
_TERM_LVCMOS_0.1_1P8  Cell operated at 1.8(nom)
|HALF_TERM_LVCMOS_0.1_1P8
|BUFFER OPERATING UNDER HALF TERMINATION MODE AND LVCMOS RECIVER MODE WITH
| 1.8V SUPPLY WITH +/-0.1V VARIATION
NOSR0_NOTERM_0.1_1P8  Cell operated at 1.8(nom)
|NOSR0_NOTERM_0.1_1P8
|BUFFER OPERATING AT FAST MODE WITH 1.8V SUPPLY WITH +/-0.1V VARIATION
SR0_NOTERM_0.1_1P8  Cell operated at 1.8(nom)
|SR0_NOTERM_0.1_1P8
|BUFFER OPERATING AT SLOW MODE WITH 1.8V SUPPLY WITH +/-0.1V VARIATION
LL_TERM_SSTL_0.1_1P8  Cell operated at 1.8(nom)
|FULL_TERM_SSTL_0.1_1P8
|BUFFER OPERATING UNDER FULL TERMINATION MODE AND SSTL RECIVER MODE WITH
| 1.8V SUPPLY WITH +/-0.1V VARIATION
NO_TERM_LVCM_0.1_1P8  Cell operated at 1.8(nom)
|NO_TERM_LVCMOS_0.1_1P8
|BUFFER OPERATING UNDER NO TERMINATION MODE AND LVCMOS RECIVER MODE WITH
| 1.8V SUPPLY WITH +/-0.1V VARIATION
FU_TERM_LVCM_0.1_1P8  Cell operated at 1.8(nom)
|FULL_TERM_LVCMOS_0.1_1P8
|BUFFER OPERATING UNDER FULL TERMINATION MODE AND LVCMOS RECIVER MODE WITH
| 1.8V SUPPLY WITH +/-0.1V VARIATION
NO_TERM_SSTL_0.1_1P8  Cell operated at 1.8(nom)
|NO_TERM_SSTL_0.1_1P8
|BUFFER OPERATING UNDER NO TERMINATION MODE AND SSTL RECIVER MODE WITH
| 1.8V SUPPLY WITH +/-0.1V VARIATION
LF_TERM_SSTL_0.1_1P5  Cell operated at 1.5(nom)
|HALF_TERM_SSTL_0.1_1P5
|BUFFER OPERATING UNDER HALF TERMINATION MODE AND SSTL RECIVER MODE WITH
| 1.5V SUPPLY WITH +/-0.1V VARIATION
NOSR0_NOTERM_0.1_1P5  Cell operated at 1.5(nom)
|NOSR0_NOTERM_0.1_1P5
|BUFFER OPERATING AT FAST MODE WITH 1.5V SUPPLY WITH +/-0.1V VARIATION
SR0_NOTERM_0.1_1P5  Cell operated at 1.5(nom)
|SR0_NOTERM_0.1_1P5
|BUFFER OPERATING AT SLOW MODE WITH 1.5V SUPPLY WITH +/-0.1V VARIATION
LL_TERM_SSTL_0.1_1P5  Cell operated at 1.5(nom)
|FULL_TERM_SSTL_0.1_1P5
|BUFFER OPERATING UNDER FULL TERMINATION MODE AND SSTL RECIVER MODE WITH
| 1.5V SUPPLY WITH +/-0.1V VARIATION
NO_TERM_SSTL_0.1_1P5  Cell operated at 1.5(nom)
| Models and submodels in the file (43): BC40C_PI_1P8 (I/O), BC40C_PI_3P3 (I/O), BC50B_!PI_LOW_1P8 (I/O), BC50B_!PI_HIGH_1P8 (I/O), BC50B_PI_1P8 (I/O), BC50B_!PI_LOW_3P3 (I/O), BC50B_!PI_HIGH_3P3 (I/O), BC50B_PI_3P3 (I/O), BC65A_!PI_LOW_3P3 (I/O), BC65A_!PI_HIGH_3P3 (I/O), BC65A_PI_3P3 (I/O), HYPOFFFBPB_PD_PU_1P8 (I/O), YPOFFFBPB_PD_PU_1P12 (Input), hs_dp (3-state), hs_dm (3-state), fs_dp (3-state), fs_dm (3-state), HALF_TERM_SSTL_1P8 (Input), HALF_TERM_LVCMOS_1P8 (Input), NOSR0_NOTERM_1P8 (I/O), SR0_NOTERM_1P8 (I/O), FULL_TERM_SSTL_1P8 (Input), NO_TERM_LVCMOS_1P8 (Input), FULL_TERM_LVCMOS_1P8 (Input), NO_TERM_SSTL_1P8 (Input), HALF_TERM_SSTL_1P5 (Input), NOSR0_NOTERM_1P5 (I/O), SR0_NOTERM_1P5 (I/O), FULL_TERM_SSTL_1P5 (Input), NO_TERM_SSTL_1P5 (Input), LF_TERM_SSTL_0.1_1P8 (Input), _TERM_LVCMOS_0.1_1P8 (Input), NOSR0_NOTERM_0.1_1P8 (I/O), SR0_NOTERM_0.1_1P8 (I/O), LL_TERM_SSTL_0.1_1P8 (Input), NO_TERM_LVCM_0.1_1P8 (Input), FU_TERM_LVCM_0.1_1P8 (Input), NO_TERM_SSTL_0.1_1P8 (Input), LF_TERM_SSTL_0.1_1P5 (Input), NOSR0_NOTERM_0.1_1P5 (I/O), SR0_NOTERM_0.1_1P5 (I/O), LL_TERM_SSTL_0.1_1P5 (Input), NO_TERM_SSTL_0.1_1P5 (Input)
